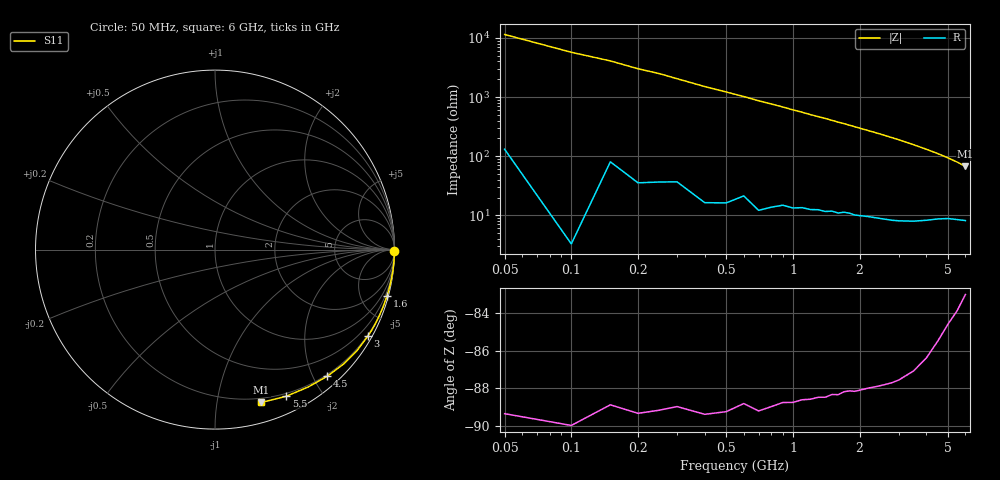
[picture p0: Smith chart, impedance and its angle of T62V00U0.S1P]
! SIEMENS Discrete & RF Semiconductors
! BAT62
! Si Schottky Diode in SOT143
! VR = 2 V
! S-Parameters:  February  1997
# GHz  S  MA  R  50
!  f  S11
! GHz  MAG  ANG
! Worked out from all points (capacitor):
!   34 points, 50 MHz to 6 GHz, reference 50 ohm
!   read as one part to ground: C = 278 fF near 50 MHz
!   lowest |Z| = 67.2 ohm at 6 GHz (marker M1)
!   S11 on the Smith chart (normalised r, x): 50 MHz: open; 1.6 GHz: 0.22, -7.54; 3 GHz: 0.16, -3.79; 4.5 GHz: 0.17, -2.21; 5.5 GHz: 0.17, -1.59; 6 GHz: 0.16, -1.33
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0.05  0.9999 -0.5
0.1  1 -1.0
0.15  0.9995 -1.4
0.2  0.9996 -1.9
0.25  0.9994 -2.3
0.4  0.9993 -3.8
0.6  0.998 -5.6
0.7  0.9984 -6.6
0.8  0.9977 -7.5
0.9  0.9968 -8.4
1  0.9964 -9.4
1.1  0.9957 -10.3
1.2  0.9951 -11.3
1.4  0.994 -13.1
1.6  0.9925 -15.1
1.7  0.9913 -16.0
2  0.9893 -19.0
2.2  0.9875 -21.0
2.4  0.9858 -23.0
2.6  0.9839 -25.1
2.8  0.9818 -27.3
3  0.9792 -29.5
3.5  0.9709 -35.4
4  0.9589 -41.7
4.5  0.9428 -48.5
5  0.9249 -55.9
5.5  0.9086 -64.0
6  0.8899 -73.2
